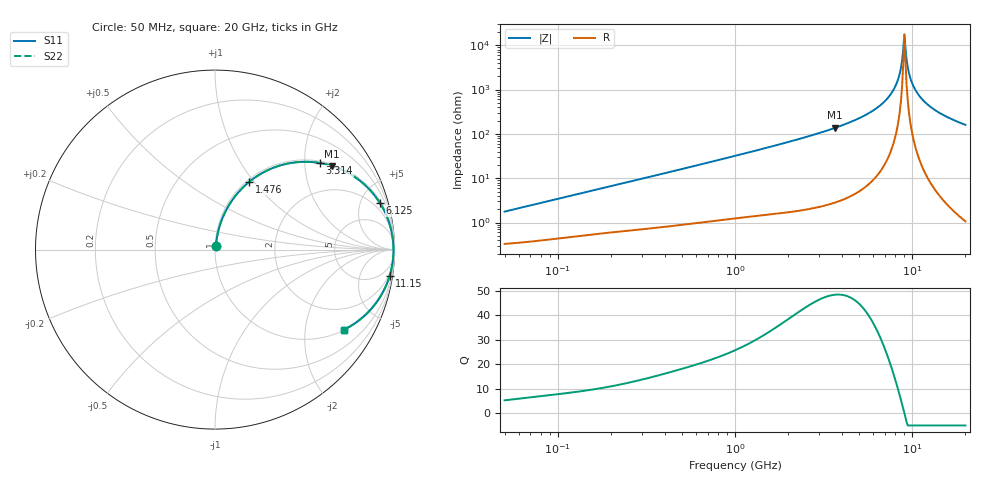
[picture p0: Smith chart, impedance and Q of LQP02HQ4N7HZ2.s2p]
!Murata Part Number: LQP02HQ4N7HZ2
!These Parameters are Measured in Series Mode Connection
!  o--[Z]--o
!Port1  Port2
!  o-------o
!Freq. Start=50[MHz] Stop=20[GHz], 401[Steps]
# Hz S RI R 50
!Freq.(Hz) S11(Real) S11(Imag) S21(Real) S21(Imag) S12(Real) S12(Imag) S22(Real) S22(Imag)
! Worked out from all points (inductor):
!   401 points, 50 MHz to 20 GHz, reference 50 ohm
!   read as one part in series: L = 5.5 nH near 51.52 MHz
!   highest Q = 48.4 at 3.681 GHz (marker M1), where L = 5.94 nH
!   self-resonance near 9.042 GHz
!   S11 on the Smith chart (normalised r, x): 50 MHz: 1.01, +0.03; 1.476 GHz: 1.03, +0.95; 3.314 GHz: 1.05, +2.38; 6.125 GHz: 1.20, +7.03; 11.15 GHz: 1, -13; 20 GHz: 1.02, -3.20
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5e7  0.00359 0.0173  0.9964 -0.0173  0.9964 -0.0173  0.00359 0.0173
1.364002e8  0.0071 0.0452  0.9929 -0.0452  0.9929 -0.0452  0.0071 0.0452
3.721004e8  0.0216 0.1168  0.9784 -0.1168  0.9784 -0.1168  0.0216 0.1168
1e9  0.1017 0.2834  0.8983 -0.2834  0.8983 -0.2834  0.1017 0.2834
1.476162e9  0.1919 0.3786  0.8081 -0.3786  0.8081 -0.3786  0.1919 0.3786
2.728004e9  0.4675 0.4879  0.5325 -0.4879  0.5325 -0.4879  0.4675 0.4879
3.314454e9  0.5854 0.4823  0.4146 -0.4823  0.4146 -0.4823  0.5854 0.4823
3.680849e9  0.6506 0.4666  0.3494 -0.4666  0.3494 -0.4666  0.6506 0.4666
4.89267e9  0.817 0.3758  0.183 -0.3758  0.183 -0.3758  0.817 0.3758
6.125241e9  0.919 0.2593  0.081 -0.2593  0.081 -0.2593  0.919 0.2593
7.442007e9  0.9746 0.1354  0.0254 -0.1354  0.0254 -0.1354  0.9746 0.1354
8.264682e9  0.9899 0.0636  0.0101 -0.0636  0.0101 -0.0636  0.9899 0.0636
8.516016e9  0.9923 0.0427  0.00773 -0.0427  0.00773 -0.0427  0.9923 0.0427
8.907419e9  0.9942 0.0112  0.00584 -0.0112  0.00584 -0.0112  0.9942 0.0112
9.041845e9  0.9943 0.000643  0.00566 -0.000643  0.00566 -0.000643  0.9943 0.000643
9.316812e9  0.994 -0.0204  0.00596 0.0204  0.00596 0.0204  0.994 -0.0204
9.600142e9  0.9928 -0.0414  0.00717 0.0414  0.00717 0.0414  0.9928 -0.0414
9.892087e9  0.9907 -0.0624  0.00927 0.0624  0.00927 0.0624  0.9907 -0.0624
1.034674e10  0.9859 -0.0936  0.0141 0.0936  0.0141 0.0936  0.9859 -0.0936
1.115139e10  0.9735 -0.1448  0.0265 0.1448  0.0265 0.1448  0.9735 -0.1448
1.417136e10  0.8988 -0.2948  0.1012 0.2948  0.1012 0.2948  0.8988 -0.2948
2e10  0.7181 -0.4466  0.2819 0.4466  0.2819 0.4466  0.7181 -0.4466
